(* Logix 5000 Routine export SpeedPlus_Program; software revision 20.01 *)

TYPE SpeedPlus_Output :
STRUCT
   SW1_Enabled : BOOL;
   SW1_Latching : BOOL;
   SW1_Failsafe : BOOL;
   SW1_on_SP1 : BOOL;
   SW1_on_SP2 : BOOL;
   SW1_on_SP3 : BOOL;
   SW1_on_RPM : BOOL;
   Reserved1 : BOOL;
   SW2_Enabled : BOOL;
   SW2_Latching : BOOL;
   SW2_Failsafe : BOOL;
   SW2_on_SP1 : BOOL;
   SW2_on_SP2 : BOOL;
   SW2_on_SP3 : BOOL;
   SW2_on_RPM : BOOL;
   Setpoints_Lockout : BOOL;
   Reserved2 : INT;
   Status_Control : INT;
   Reserved3 : INT;
END_STRUCT
END_TYPE

TYPE Key_Command :
STRUCT
   Command : SINT;
   Compliment : SINT;
   Arg_1 : SINT;
   Arg_2 : SINT;
END_STRUCT
END_TYPE

TYPE SpeedPlus_Data :
STRUCT
   Reconfigure : BOOL;
   Start_SP1 : BOOL;
   Start_SP2 : BOOL;
   Start_SP3 : BOOL;
   Start_ALL_SPs : BOOL;
   Unlatch_Switches : BOOL;
   Unlatch_SW1 : BOOL;
   Unlatch_SW2 : BOOL;
   Device_Reset : BOOL;
   Keycommand_ONS : BOOL; {access Read Only}
   Reconfigure_ONS : BOOL; {access Read Only}
   KCMD : SINT; {access Read Only}
   CMD_ARG : SINT; {access Read Only}
   GT_Backup : INT; {access Read Only}
   MaxRPM_Backup : DINT; {access Read Only}
   Ratio_Backup : REAL; {access Read Only}
   Output_Current_Scaled : REAL; {access Read Only}
   Supply_Voltage_Scaled : REAL; {access Read Only}
   Key_Command : Key_Command; {access Read Only}
   Status : Communication_Status;
END_STRUCT
END_TYPE

TYPE SpeedPlus_Input :
STRUCT
   SW1_Enabled_Echo : BOOL;
   SW1_Latching_Echo : BOOL;
   SW1_Failsafe_Echo : BOOL;
   SW1_on_SP1_Echo : BOOL;
   SW1_on_SP2_Echo : BOOL;
   SW1_on_SP3_Echo : BOOL;
   SW1_on_RPM_Echo : BOOL;
   Output_Reserved1_Echo : BOOL;
   SW2_Enabled_Echo : BOOL;
   SW2_Latching_Echo : BOOL;
   SW2_Failsafe_Echo : BOOL;
   SW2_on_SP1_Echo : BOOL;
   SW2_on_SP2_Echo : BOOL;
   SW2_on_SP3_Echo : BOOL;
   SW2_on_RPM_Echo : BOOL;
   Setpoints_Lockout_Echo : BOOL;
   DI_Active : BOOL;
   DI_Reserved_Active : BOOL;
   SP1_Active : BOOL;
   SP2_Active : BOOL;
   SP3_Active : BOOL;
   Reserved1 : BOOL;
   Current_Loop_Faulted : BOOL;
   Current_Loop_Output_Out_of_Range : BOOL;
   Digital_Out_1_Active : BOOL;
   Digital_Out_2_Active : BOOL;
   SP1_Tripped : BOOL;
   SP2_Tripped : BOOL;
   SP3_Tripped : BOOL;
   Rotating : BOOL;
   Reserved2 : BOOL;
   Supply_Voltage_Fault : BOOL;
   Output_Reserved2_Echo : INT;
   Loop_Output : INT;
   Speed_Unfiltered : REAL;
   Accelleration : INT;
   Supply_Voltage : INT;
   Speed : DINT;
   Status : INT;
   Output_Reserved3_Echo : INT;
END_STRUCT
END_TYPE

TYPE Communication_Status :
STRUCT
   Count : INT; {access Read Only}
   Status : INT; {access Read Only}
END_STRUCT
END_TYPE

VAR_GLOBAL   (* controller tags *)
   SpeedPlus_Input : SpeedPlus_Input := (SW1_Enabled_Echo := 1, SW1_on_SP1_Echo := 1, SW1_on_SP2_Echo := 1, SW2_Enabled_Echo := 1, SW2_Latching_Echo := 1, SW2_Failsafe_Echo := 1, SW2_on_SP3_Echo := 1, SP1_Active := 1, SP2_Active := 1, SP3_Active := 1, Rotating := 1, Loop_Output := 499, Speed_Unfiltered := 499.8, Supply_Voltage := 230, Speed := 500); {access Read Only}
   SpeedPlus_Program_Data : SpeedPlus_Data := (GT_Backup := 60, MaxRPM_Backup := 2400, Ratio_Backup := 1.0, Output_Current_Scaled := 4.99, Supply_Voltage_Scaled := 23.0, Key_Command.Compliment := -4);
   SpeedPlus_KeyCommand : MESSAGE;
        MessageParameters(MessageType := CIP Generic, RequestedLength := 4, ConnectedFlag := 2, ConnectionPath := SpeedPlus, ServiceCode := 16#004b, ObjectType := 16#0070, TargetObject := 1, LocalElement := SpeedPlus_Program_Data.Key_Command.Command)
   SpeedPlus_Output : SpeedPlus_Output := (SW1_Enabled := 1, SW1_on_SP1 := 1, SW1_on_SP2 := 1, SW2_Enabled := 1, SW2_Latching := 1, SW2_Failsafe := 1, SW2_on_SP3 := 1);
   SpeedPlus_Reconfigure : MESSAGE;
        MessageParameters(MessageType := Module Reconfigure, RequestedLength := 1, ConnectionPath := SpeedPlus)
END_VAR

PROGRAM DET_COM

ROUTINE SpeedPlus_Program   (* ladder *)
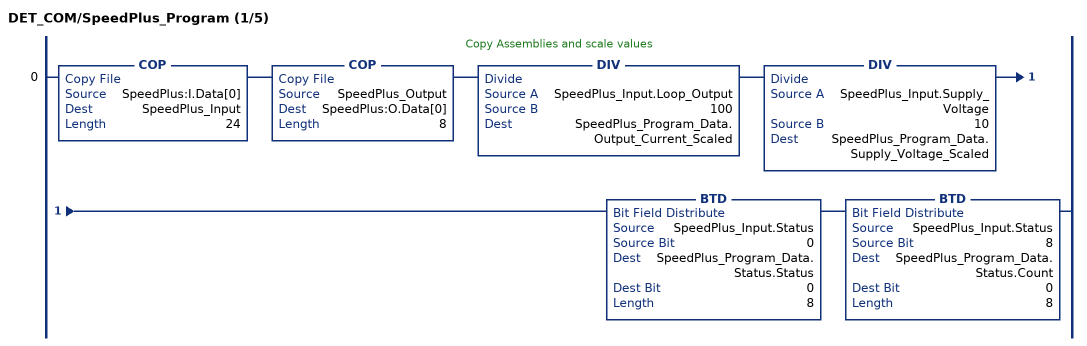
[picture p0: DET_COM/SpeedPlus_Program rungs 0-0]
   // Copy Assemblies and scale values
   0: COP(SpeedPlus:I.Data[0],SpeedPlus_Input,24)COP(SpeedPlus_Output,SpeedPlus:O.Data[0],8)DIV(SpeedPlus_Input.Loop_Output,100,SpeedPlus_Program_Data.Output_Current_Scaled)DIV(SpeedPlus_Input.Supply_Voltage,10,SpeedPlus_Program_Data.Supply_Voltage_Scaled)BTD(SpeedPlus_Input.Status,0,SpeedPlus_Program_Data.Status.Status,0,8)BTD(SpeedPlus_Input.Status,8,SpeedPlus_Program_Data.Status.Count,0,8);
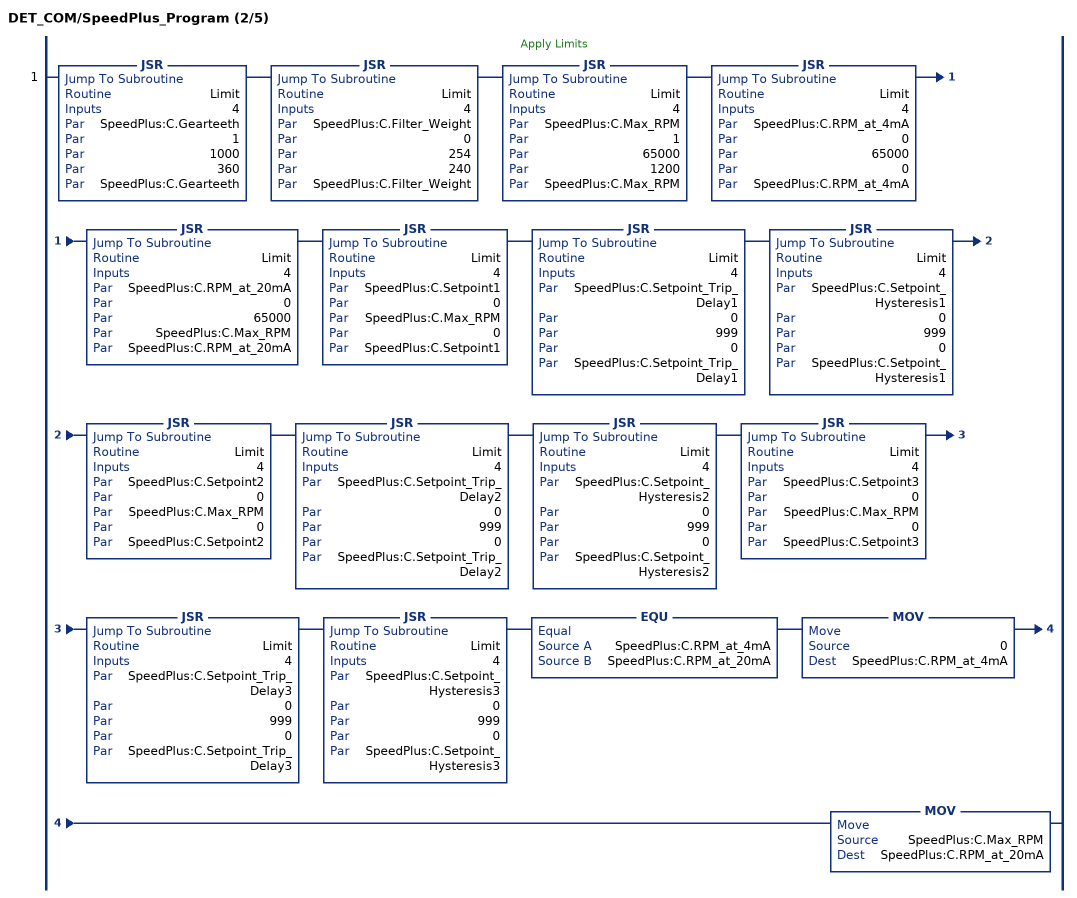
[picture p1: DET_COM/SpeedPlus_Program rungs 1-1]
   // Apply Limits
   1: JSR(Limit,4,SpeedPlus:C.Gearteeth,1,1000,360,SpeedPlus:C.Gearteeth)JSR(Limit,4,SpeedPlus:C.Filter_Weight,0,254,240,SpeedPlus:C.Filter_Weight)JSR(Limit,4,SpeedPlus:C.Max_RPM,1,65000,1200,SpeedPlus:C.Max_RPM)JSR(Limit,4,SpeedPlus:C.RPM_at_4mA,0,65000,0,SpeedPlus:C.RPM_at_4mA)JSR(Limit,4,SpeedPlus:C.RPM_at_20mA,0,65000,SpeedPlus:C.Max_RPM,SpeedPlus:C.RPM_at_20mA)JSR(Limit,4,SpeedPlus:C.Setpoint1,0,SpeedPlus:C.Max_RPM,0,SpeedPlus:C.Setpoint1)JSR(Limit,4,SpeedPlus:C.Setpoint_Trip_Delay1,0,999,0,SpeedPlus:C.Setpoint_Trip_Delay1)JSR(Limit,4,SpeedPlus:C.Setpoint_Hysteresis1,0,999,0,SpeedPlus:C.Setpoint_Hysteresis1)JSR(Limit,4,SpeedPlus:C.Setpoint2,0,SpeedPlus:C.Max_RPM,0,SpeedPlus:C.Setpoint2)JSR(Limit,4,SpeedPlus:C.Setpoint_Trip_Delay2,0,999,0,SpeedPlus:C.Setpoint_Trip_Delay2)JSR(Limit,4,SpeedPlus:C.Setpoint_Hysteresis2,0,999,0,SpeedPlus:C.Setpoint_Hysteresis2)JSR(Limit,4,SpeedPlus:C.Setpoint3,0,SpeedPlus:C.Max_RPM,0,SpeedPlus:C.Setpoint3)JSR(Limit,4,SpeedPlus:C.Setpoint_Trip_Delay3,0,999,0,SpeedPlus:C.Setpoint_Trip_Delay3)JSR(Limit,4,SpeedPlus:C.Setpoint_Hysteresis3,0,999,0,SpeedPlus:C.Setpoint_Hysteresis3)EQU(SpeedPlus:C.RPM_at_4mA,SpeedPlus:C.RPM_at_20mA)MOV(0,SpeedPlus:C.RPM_at_4mA)MOV(SpeedPlus:C.Max_RPM,SpeedPlus:C.RPM_at_20mA);
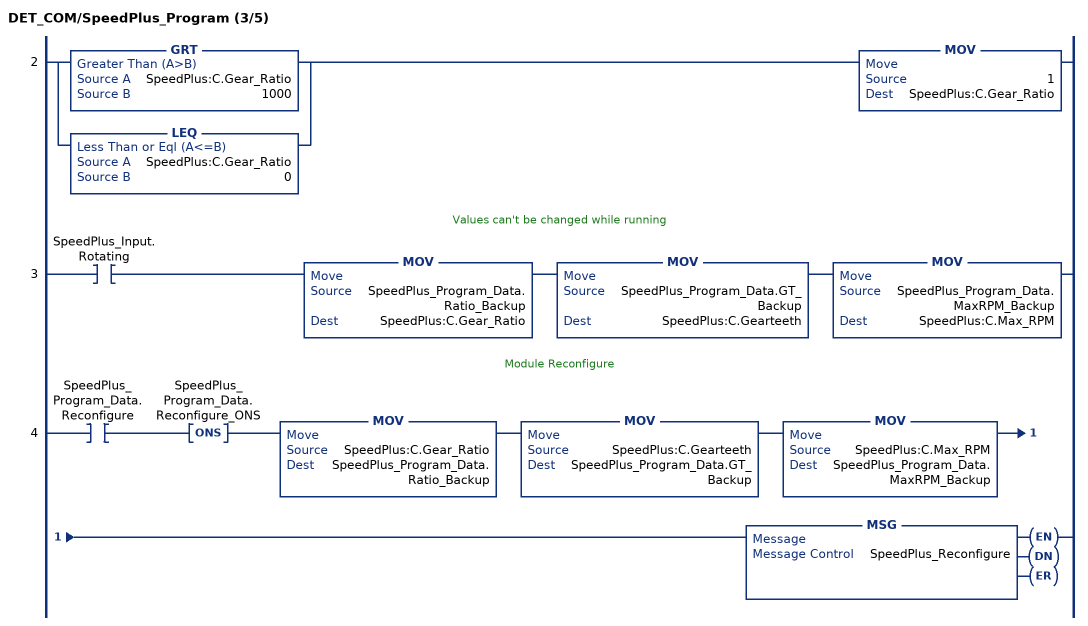
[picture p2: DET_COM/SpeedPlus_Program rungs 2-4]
   2: [GRT(SpeedPlus:C.Gear_Ratio,1000) ,LEQ(SpeedPlus:C.Gear_Ratio,0) ]MOV(1,SpeedPlus:C.Gear_Ratio);
   // Values can't be changed while running
   3: XIC(SpeedPlus_Input.Rotating)MOV(SpeedPlus_Program_Data.Ratio_Backup,SpeedPlus:C.Gear_Ratio)MOV(SpeedPlus_Program_Data.GT_Backup,SpeedPlus:C.Gearteeth)MOV(SpeedPlus_Program_Data.MaxRPM_Backup,SpeedPlus:C.Max_RPM);
   // Module Reconfigure
   4: XIC(SpeedPlus_Program_Data.Reconfigure)ONS(SpeedPlus_Program_Data.Reconfigure_ONS)MOV(SpeedPlus:C.Gear_Ratio,SpeedPlus_Program_Data.Ratio_Backup)MOV(SpeedPlus:C.Gearteeth,SpeedPlus_Program_Data.GT_Backup)MOV(SpeedPlus:C.Max_RPM,SpeedPlus_Program_Data.MaxRPM_Backup)MSG(SpeedPlus_Reconfigure);
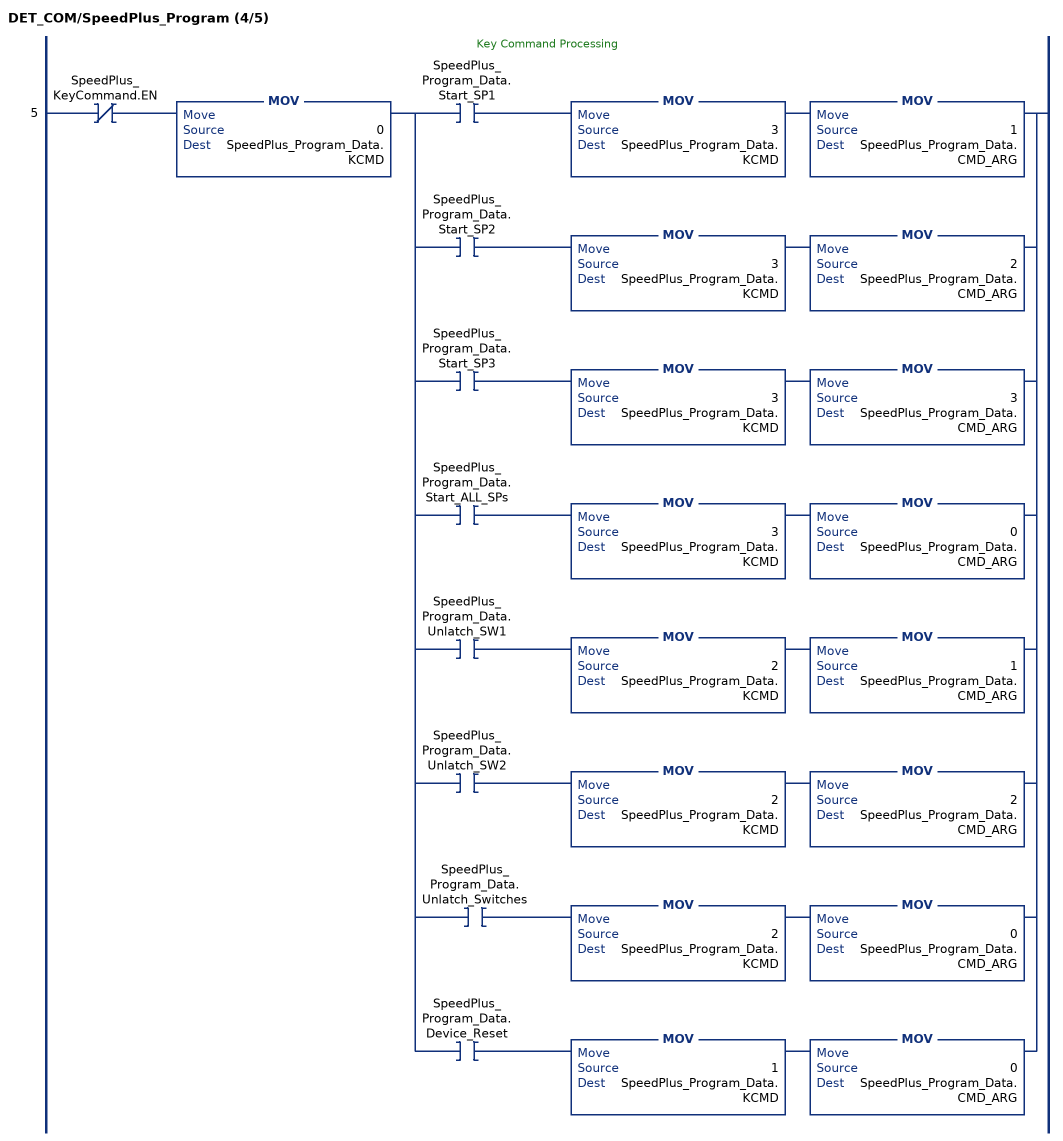
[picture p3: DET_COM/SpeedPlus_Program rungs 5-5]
   // Key Command Processing
   5: XIO(SpeedPlus_KeyCommand.EN)MOV(0,SpeedPlus_Program_Data.KCMD)[XIC(SpeedPlus_Program_Data.Start_SP1) MOV(3,SpeedPlus_Program_Data.KCMD) MOV(1,SpeedPlus_Program_Data.CMD_ARG) ,XIC(SpeedPlus_Program_Data.Start_SP2) MOV(3,SpeedPlus_Program_Data.KCMD) MOV(2,SpeedPlus_Program_Data.CMD_ARG) ,XIC(SpeedPlus_Program_Data.Start_SP3) MOV(3,SpeedPlus_Program_Data.KCMD) MOV(3,SpeedPlus_Program_Data.CMD_ARG) ,XIC(SpeedPlus_Program_Data.Start_ALL_SPs) MOV(3,SpeedPlus_Program_Data.KCMD) MOV(0,SpeedPlus_Program_Data.CMD_ARG) ,XIC(SpeedPlus_Program_Data.Unlatch_SW1) MOV(2,SpeedPlus_Program_Data.KCMD) MOV(1,SpeedPlus_Program_Data.CMD_ARG) ,XIC(SpeedPlus_Program_Data.Unlatch_SW2) MOV(2,SpeedPlus_Program_Data.KCMD) MOV(2,SpeedPlus_Program_Data.CMD_ARG) ,XIC(SpeedPlus_Program_Data.Unlatch_Switches) MOV(2,SpeedPlus_Program_Data.KCMD) MOV(0,SpeedPlus_Program_Data.CMD_ARG) ,XIC(SpeedPlus_Program_Data.Device_Reset) MOV(1,SpeedPlus_Program_Data.KCMD) MOV(0,SpeedPlus_Program_Data.CMD_ARG) ];
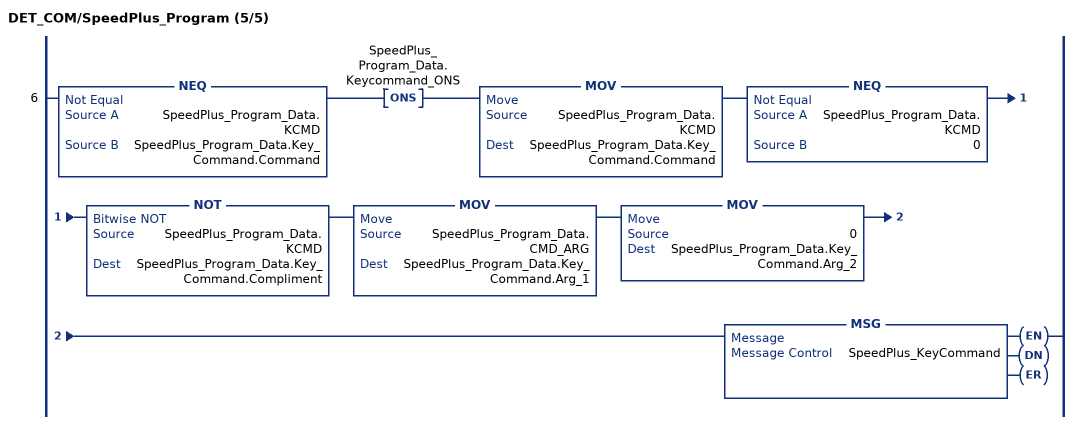
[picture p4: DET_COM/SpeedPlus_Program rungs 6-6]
   6: NEQ(SpeedPlus_Program_Data.KCMD,SpeedPlus_Program_Data.Key_Command.Command)ONS(SpeedPlus_Program_Data.Keycommand_ONS)MOV(SpeedPlus_Program_Data.KCMD,SpeedPlus_Program_Data.Key_Command.Command)NEQ(SpeedPlus_Program_Data.KCMD,0)NOT(SpeedPlus_Program_Data.KCMD,SpeedPlus_Program_Data.Key_Command.Compliment)MOV(SpeedPlus_Program_Data.CMD_ARG,SpeedPlus_Program_Data.Key_Command.Arg_1)MOV(0,SpeedPlus_Program_Data.Key_Command.Arg_2)MSG(SpeedPlus_KeyCommand);
END_ROUTINE
END_PROGRAM
